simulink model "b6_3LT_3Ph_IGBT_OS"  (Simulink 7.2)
settings: Solver=ode3  SolverMode=SingleTasking  StartTime=0.0  StopTime=0.1  FixedStep=10e-6  MaxStep=1e-5  RelTol=1e-4  AbsTol=1e-4
PreLoadFcn:
  | INIT_B6_3L_3Ph_IGBT_OS
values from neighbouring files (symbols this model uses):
  C = 10e-3*1    (= 0.01)    [INIT_B6_2L_3Ph_IGBT_OS.m]    (also in INIT_B6_3L_3Ph_IGBT_OS.m; INIT_MMC_100L.m = 0.005; INIT_MMC_200L.m = 0.005; INIT_MMC_20L.m)
  FS = 900    [INIT_B6_2L_3Ph_IGBT_OS.m]    (also in INIT_B6_3L_3Ph_IGBT_OS.m; INIT_PWM_2L.m = 1000; INIT_PWM_3L.m = 1000; INIT_PWM_Con.m = 1000)
  I_B = INS    [INIT_B6_2L_3Ph_IGBT_OS.m]    (also in INIT_B6_3L_3Ph_IGBT_OS.m; INIT_PWM_2L.m = INP; INIT_PWM_3L.m = INP; INIT_PWM_Con.m = INP)
  IDC = PDC/VDC    (= 166.666666667)    [INIT_B6_2L_3Ph_IGBT_OS.m]    (also in INIT_B6_3L_3Ph_IGBT_OS.m = 100; INIT_PWM_2L.m = 16.6666666667; INIT_PWM_3L.m = 83.3333333333; INIT_PWM_Con.m = 83.3333333333)
  LS = 1e-3    (= 0.001)    [INIT_B6_2L_3Ph_IGBT_OS.m]    (also in INIT_B6_3L_3Ph_IGBT_OS.m; INIT_MMC_100L.m = 0.025; INIT_MMC_200L.m = 0.025; INIT_MMC_20L.m = 0.0025)
  UC0 = 600    [INIT_B6_2L_3Ph_IGBT_OS.m]    (also in INIT_B6_3L_3Ph_IGBT_OS.m = 500; INIT_MMC_100L.m = 6800; INIT_MMC_200L.m = 3400; INIT_MMC_20L.m = 5000)
  UNS = ULLP/sqrt(3)    [INIT_B6_2L_3Ph_IGBT_OS.m]    (also in INIT_B6_3L_3Ph_IGBT_OS.m; INIT_MMC_100L.m = ULLP/sqrt(3)*340/400; INIT_MMC_200L.m = ULLP/sqrt(3)*340/400; INIT_MMC_20L.m)

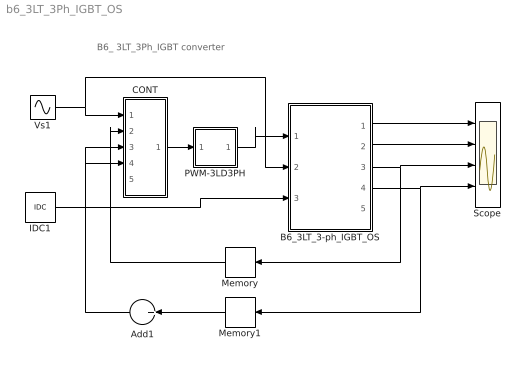
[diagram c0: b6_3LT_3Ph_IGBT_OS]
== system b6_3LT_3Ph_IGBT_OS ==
  note: B6_ 3LT_3Ph_IGBT converter
  Add1 : Sum  Orientation=left  Inputs=+  OutDataType=sfix(16)  OutScaling=2^-10
  B6_3LT_3-ph_IGBT_OS : Subsystem  mask(6-Pulse 3-LT IGBT 3-Phase Converter){LS=LS, C=C, VC0=UC0, RL=1e6}
      mask prompts: LS "Source Inductance"; C "Load Cap"; VC0 "Initial Cap Voltage"; RL "Load Resistance"
      mask help: Input Vector u: u[0]= IGBT1.gate u[1]= IGBT2.gate u[2]= IGBT3.gate u[3]= IGBT4.gate u[4]= IGBT5.gate u[5]= IGBT6.gate u[6]= IGBT7.gate u[7]= IGBT8.gate u[8]= IGBT9.gate u[9]= IGBT10.gate u[10]= IGBT11.gate u[11]= IGBT12.gate u[12]= V1.V u[13]= V2.V u[14]= V3.V u[15]= IDC.i Output Vector y: y[0]= T1.I y[1]= D1.I y[2]= T1.V y[3]= T2.I y[4]= D2.I y[5]= T2.V y[6]= LS1.I y[7]= LS2.I y[8]= LS3.I y[9]= DC1.V y[10]= DC2.V y[11]= Vab.V Parameter Vector p: p[0]= Ls.L p[1]= C1.C p[2]= C1.vC0 p[3]= R1.r You can pause the simulation during running, change the Parameters you want and continue the Simulation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
  CONT : Subsystem
  IDC1 : Constant  Value=IDC
  Memory : Memory  Orientation=left
  Memory1 : Memory  Orientation=left
  PWM-3LD3PH : Subsystem  mask(PWM-3LD3PH){FT=FS, PHT=0, A=0.5, O1=0.5, O2=-0.5, DT=1e-6}
      mask prompts: FT "Frequency of Trian Sig."; PHT "Phase Angle of Trian. Sig."; A "Amplitude of Trian. Sig."; O1 "Offset of 1st Trian"; O2 "Offset of 2nd Trian."; DT "Dead Time"
      mask help: Pulse Width Modulation for 3 Phase 3 Level Neutral point clamped Converter
  Scope : Scope  NumInputPorts=4
  Vs1 : Sin  Amplitude=UNS  Frequency=50*2*pi  Phase="[0  -2*pi/3   -4*pi/3]"  SampleTime=0
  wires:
  Vs1/1 -> CONT/1(UN), B6_3LT_3-ph_IGBT_OS/2(vS)
  IDC1/1 -> CONT/4(Id*), B6_3LT_3-ph_IGBT_OS/3(iDC)
  CONT/1(A) -> PWM-3LD3PH/1(In1)
  PWM-3LD3PH/1(Out1) -> B6_3LT_3-ph_IGBT_OS/1(SWs)
  B6_3LT_3-ph_IGBT_OS/3(iLs123) -> Scope/3, Memory/1
  Memory/1 -> CONT/2(Iwr)
  B6_3LT_3-ph_IGBT_OS/1(iT1,iD1,vT1) -> Scope/1
  B6_3LT_3-ph_IGBT_OS/2(iT2,iD2,vT2) -> Scope/2
  B6_3LT_3-ph_IGBT_OS/4(vDC12) -> Scope/4, Memory1/1
  Memory1/1 -> Add1/1
  Add1/1 -> CONT/3(UDC)

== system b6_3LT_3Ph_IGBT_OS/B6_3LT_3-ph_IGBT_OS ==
  SWs : Inport  OutDataType=sfix(16)  OutScaling=2^0
  vS : Inport  Port=2  OutDataType=sfix(16)  OutScaling=2^0
  iDC : Inport  Port=3  OutDataType=sfix(16)  OutScaling=2^0
  Mux : Mux  Inputs="[12  3  1]"
  b2_IGBT : S-Function  FunctionName=s_b6_3LT_3Ph_IGBT_OS  Parameters="[ LS  C  VC0 RL]"  EnableBusSupport=off
  iT1,iD1,vT1 : Outport  OutDataType=sfix(16)  OutScaling=2^0
  iT2,iD2,vT2 : Outport  Port=2  OutDataType=sfix(16)  OutScaling=2^0
  iLs123 : Outport  Port=3  OutDataType=sfix(16)  OutScaling=2^0
  vDC12 : Outport  Port=4  OutDataType=sfix(16)  OutScaling=2^0
  vab : Outport  Port=5  OutDataType=sfix(16)  OutScaling=2^0
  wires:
  b2_IGBT/5 -> vab/1
  SWs/1 -> Mux/1
  vS/1 -> Mux/2
  b2_IGBT/1 -> iT1,iD1,vT1/1
  b2_IGBT/2 -> iT2,iD2,vT2/1
  b2_IGBT/3 -> iLs123/1
  iDC/1 -> Mux/3
  Mux/1 -> b2_IGBT/1
  b2_IGBT/4 -> vDC12/1

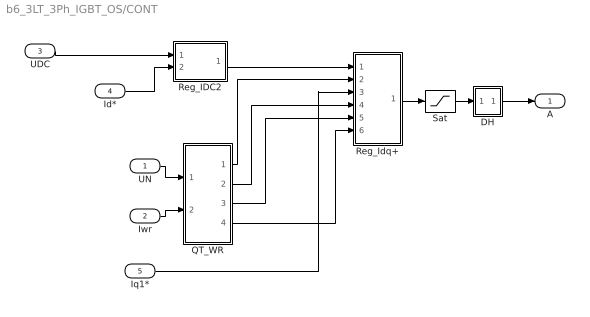
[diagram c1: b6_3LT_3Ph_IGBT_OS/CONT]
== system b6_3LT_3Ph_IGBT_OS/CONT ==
  UN : Inport
  Iwr : Inport  Port=2
  UDC : Inport  Port=3
  Id* : Inport  Port=4
  Iq1* : Inport  Port=5
  DH : Subsystem
  QT_WR : Subsystem
  Reg_IDC2 : Subsystem
  Reg_Idq+ : Subsystem
  Sat : Saturate  UpperLimit=1.5  LowerLimit=-1.5
  A : Outport
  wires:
  Sat/1 -> DH/1(I)
  Reg_Idq+/1(A+) -> Sat/1
  Id*/1 -> Reg_IDC2/2(Id*)
  DH/1(O) -> A/1
  UDC/1 -> Reg_IDC2/1(UDC)
  UN/1 -> QT_WR/1(UN)
  Iwr/1 -> QT_WR/2(I_WR)
  Reg_IDC2/1(Id1*) -> Reg_Idq+/1(Id1*)
  QT_WR/3(th1) -> Reg_Idq+/5(th)
  Iq1*/1 -> Reg_Idq+/3(Iq1*)
  QT_WR/2(Iq1) -> Reg_Idq+/4(Iq1)
  QT_WR/1(Id1) -> Reg_Idq+/2(Id1)
  QT_WR/4(Ud) -> Reg_Idq+/6(Ud)

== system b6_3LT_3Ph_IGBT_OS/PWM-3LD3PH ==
  In1 : Inport  OutDataType=sfix(16)  OutScaling=2^0
  Demux1 : Demux  Outputs=3
  Mux1 : Mux  Inputs=3
  PWM-3LD1PH : Subsystem  mask(PWM-3LD_1PH){FT=FT, PHT=PHT, A=A, O1=O1, O2=O2, DT=DT}
      mask prompts: FT "Frequency of Trian Sig."; PHT "Phase Angle of Trian. Sig."; A "Amplitude of Trian. Sig."; O1 "Offset of 1st Trian"; O2 "Offset of 2nd Trian."; DT "Dead Time"
      mask help: Pulse Width Modulation for 1 Leg of 3 Level Neutral point clamped Converter
  PWM-3LD1PH1 : Subsystem  mask(PWM-3LD_1PH){FT=FT, PHT=PHT, A=A, O1=O1, O2=O2, DT=DT}
      mask prompts: FT "Frequency of Trian Sig."; PHT "Phase Angle of Trian. Sig."; A "Amplitude of Trian. Sig."; O1 "Offset of 1st Trian"; O2 "Offset of 2nd Trian."; DT "Dead Time"
      mask help: Pulse Width Modulation for 1 Leg of 3 Level Neutral point clamped Converter
  PWM-3LD1PH2 : Subsystem  mask(PWM-3LD_1PH){FT=FT, PHT=PHT, A=A, O1=O1, O2=O2, DT=DT}
      mask prompts: FT "Frequency of Trian Sig."; PHT "Phase Angle of Trian. Sig."; A "Amplitude of Trian. Sig."; O1 "Offset of 1st Trian"; O2 "Offset of 2nd Trian."; DT "Dead Time"
      mask help: Pulse Width Modulation for 1 Leg of 3 Level Neutral point clamped Converter
  Out1 : Outport
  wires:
  In1/1 -> Demux1/1
  Demux1/3 -> PWM-3LD1PH2/1(In1)
  Demux1/2 -> PWM-3LD1PH1/1(In1)
  Demux1/1 -> PWM-3LD1PH/1(In1)
  Mux1/1 -> Out1/1
  PWM-3LD1PH2/1(Out1) -> Mux1/3
  PWM-3LD1PH1/1(Out1) -> Mux1/2
  PWM-3LD1PH/1(Out1) -> Mux1/1

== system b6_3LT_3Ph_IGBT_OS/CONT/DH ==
  I : Inport
  Gain : Gain  Gain=0.5
  MinMax : MinMax
  MinMax1 : MinMax  Function=max
  Sum6 : Sum  Inputs=--
  Sum7 : Sum
  O : Outport  InitialOutput=0
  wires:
  I/1 -> MinMax1/1, MinMax/1, Sum7/1
  MinMax/1 -> Sum6/1
  MinMax1/1 -> Sum6/2
  Sum6/1 -> Gain/1
  Gain/1 -> Sum7/2
  Sum7/1 -> O/1

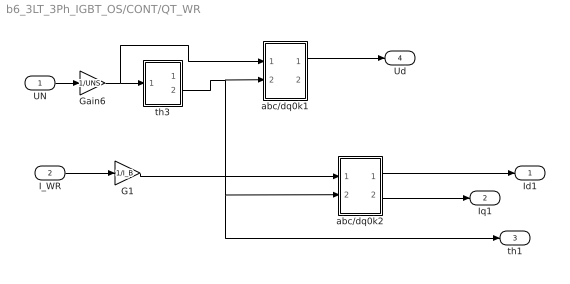
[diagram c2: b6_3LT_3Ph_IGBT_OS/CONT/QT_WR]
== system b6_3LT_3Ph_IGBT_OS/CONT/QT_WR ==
  UN : Inport
  I_WR : Inport  Port=2
  G1 : Gain  Gain=1/I_B
  Gain6 : Gain  Gain=1/UNS
  abc/dq0k1 : Subsystem
  abc/dq0k2 : Subsystem
  th3 : Subsystem
  Id1 : Outport
  Iq1 : Outport  Port=2
  th1 : Outport  Port=3
  Ud : Outport  Port=4
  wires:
  th3/2(th) -> abc/dq0k2/2(th), th1/1, abc/dq0k1/2(th)
  I_WR/1 -> G1/1
  G1/1 -> abc/dq0k2/1(a)
  UN/1 -> Gain6/1
  Gain6/1 -> th3/1(abc), abc/dq0k1/1(a)
  abc/dq0k2/1(dk) -> Id1/1
  abc/dq0k2/2(qk) -> Iq1/1
  abc/dq0k1/1(dk) -> Ud/1

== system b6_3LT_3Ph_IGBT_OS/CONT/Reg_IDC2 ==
  UDC : Inport
  Id* : Inport  Port=2
  Add : Sum
  G1 : Gain  Gain=1/IDC
  G4 : Gain  Gain=1/2/UC0
  PIC : Subsystem  mask(PI-controller){Kp=2, Ki=10, lim=2, Ts=-1}
      mask prompts: Kp "Proportional gain (Kp)"; Ki "Integral gain (Ki)"; lim "Output limit"; Ts "Sampling time (s)"
      mask help: Proportional-Integral Controller
  Sat : Saturate  UpperLimit=2  LowerLimit=-2
  UDC* : Constant  Value=1.0
  Id1* : Outport
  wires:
  Id*/1 -> G1/1
  PIC/1(e*) -> Add/2
  Sat/1 -> Id1*/1
  Add/1 -> Sat/1
  G4/1 -> PIC/2(c)
  UDC*/1 -> PIC/1(c*)
  UDC/1 -> G4/1
  G1/1 -> Add/1

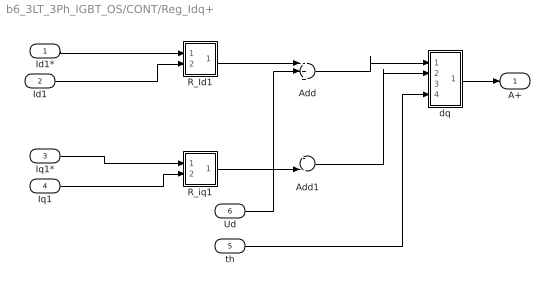
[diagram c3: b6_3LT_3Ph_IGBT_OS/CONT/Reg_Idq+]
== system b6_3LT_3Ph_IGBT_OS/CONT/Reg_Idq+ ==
  Id1* : Inport
  Id1 : Inport  Port=2
  Iq1* : Inport  Port=3
  Iq1 : Inport  Port=4
  th : Inport  Port=5
  Ud : Inport  Port=6
  Add : Sum  Inputs=-++
  Add1 : Sum  Inputs=--
  R_Id1 : Subsystem  mask(PI-controller){Kp=0.1, Ki=200, lim=2, Ts=-1}
      mask prompts: Kp "Proportional gain (Kp)"; Ki "Integral gain (Ki)"; lim "Output limit"; Ts "Sampling time (s)"
      mask help: Proportional-Integral Controller
  R_iq1 : Subsystem  mask(PI-controller){Kp=0.1, Ki=200, lim=2, Ts=-2}
      mask prompts: Kp "Proportional gain (Kp)"; Ki "Integral gain (Ki)"; lim "Output limit"; Ts "Sampling time (s)"
      mask help: Proportional-Integral Controller
  dq : Subsystem
  A+ : Outport
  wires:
  Iq1/1 -> R_iq1/2(c)
  Iq1*/1 -> R_iq1/1(c*)
  Id1/1 -> R_Id1/2(c)
  Id1*/1 -> R_Id1/1(c*)
  dq/1(a) -> A+/1
  th/1 -> dq/4(th)
  R_Id1/1(e*) -> Add/1
  R_iq1/1(e*) -> Add1/2
  Add/1 -> dq/1(dk)
  Add1/1 -> dq/2(qk)
  Ud/1 -> Add/2

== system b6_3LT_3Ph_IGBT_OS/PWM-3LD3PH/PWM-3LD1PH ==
  In1 : Inport  OutDataType=sfix(16)  OutScaling=2^0
  Mux : Mux
  SS : Subsystem
  SS1 : Subsystem
  Out1 : Outport
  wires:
  In1/1 -> SS1/1(I1), SS/1(I1)
  SS1/1(O1) -> Mux/2
  SS/2(O2) -> Mux/3
  Mux/1 -> Out1/1
  SS/1(O1) -> Mux/1
  SS1/2(O2) -> Mux/4

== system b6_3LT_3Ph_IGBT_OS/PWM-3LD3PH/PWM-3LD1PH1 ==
  In1 : Inport  OutDataType=sfix(16)  OutScaling=2^0
  Mux : Mux
  SS : Subsystem
  SS1 : Subsystem
  Out1 : Outport
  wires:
  SS1/2(O2) -> Mux/4
  SS/1(O1) -> Mux/1
  Mux/1 -> Out1/1
  SS/2(O2) -> Mux/3
  SS1/1(O1) -> Mux/2
  In1/1 -> SS/1(I1), SS1/1(I1)

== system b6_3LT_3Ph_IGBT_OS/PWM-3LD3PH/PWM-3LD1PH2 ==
  In1 : Inport  OutDataType=sfix(16)  OutScaling=2^0
  Mux : Mux
  SS : Subsystem
  SS1 : Subsystem
  Out1 : Outport
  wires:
  In1/1 -> SS1/1(I1), SS/1(I1)
  SS1/1(O1) -> Mux/2
  SS/2(O2) -> Mux/3
  Mux/1 -> Out1/1
  SS/1(O1) -> Mux/1
  SS1/2(O2) -> Mux/4

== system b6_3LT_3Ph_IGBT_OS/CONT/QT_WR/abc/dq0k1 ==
  a : Inport
  th : Inport  Port=2
  Demux : Demux  Outputs=3
  Fcn : Fcn  Expr=u(1)*cos(u(3)) + u(2)*sin(u(3))
  Fcn1 : Fcn  Expr=-u(1)*sin(u(3)) + u(2)*cos(u(3))
  K : Gain  Gain="2/3*[1   -.5   -.5;  0   sqrt(3)/2   -sqrt(3)/2;  .5    .5    .5]"  Multiplication=Matrix(K*u)
  Mux1 : Mux  Inputs=3
  dk : Outport
  qk : Outport  Port=2
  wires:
  Demux/2 -> Mux1/2
  Demux/1 -> Mux1/1
  th/1 -> Mux1/3
  Fcn1/1 -> qk/1
  Fcn/1 -> dk/1
  Mux1/1 -> Fcn/1, Fcn1/1
  a/1 -> K/1
  K/1 -> Demux/1

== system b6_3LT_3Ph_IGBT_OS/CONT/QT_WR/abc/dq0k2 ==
  a : Inport
  th : Inport  Port=2
  Demux : Demux  Outputs=3
  Fcn : Fcn  Expr=u(1)*cos(u(3)) + u(2)*sin(u(3))
  Fcn1 : Fcn  Expr=-u(1)*sin(u(3)) + u(2)*cos(u(3))
  K : Gain  Gain="2/3*[1   -.5   -.5;  0   sqrt(3)/2   -sqrt(3)/2;  .5    .5    .5]"  Multiplication=Matrix(K*u)
  Mux1 : Mux  Inputs=3
  dk : Outport
  qk : Outport  Port=2
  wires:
  K/1 -> Demux/1
  a/1 -> K/1
  Mux1/1 -> Fcn1/1, Fcn/1
  Fcn/1 -> dk/1
  Fcn1/1 -> qk/1
  th/1 -> Mux1/3
  Demux/1 -> Mux1/1
  Demux/2 -> Mux1/2

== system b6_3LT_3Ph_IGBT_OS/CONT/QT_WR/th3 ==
  abc : Inport
  C : ComplexToMagnitudeAngle
  Demux : Demux  Outputs=3
  K : Gain  Gain="2/3*[1   -.5   -.5;  0   sqrt(3)/2   -sqrt(3)/2;  .5    .5    .5]"  Multiplication=Matrix(K*u)
  R : RealImagToComplex
  |u| : Outport
  th : Outport  Port=2
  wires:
  C/2 -> th/1
  R/1 -> C/1
  Demux/2 -> R/2
  Demux/1 -> R/1
  abc/1 -> K/1
  K/1 -> Demux/1
  C/1 -> |u|/1

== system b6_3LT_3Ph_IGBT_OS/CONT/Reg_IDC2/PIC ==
  c* : Inport  OutDataType=sfix(16)  OutScaling=2^0
  c : Inport  Port=2  OutDataType=sfix(16)  OutScaling=2^0
  Gain : Gain  Gain=Ki  ParameterDataType=sfix(16)  ParameterScaling=2^0  OutDataType=sfix(16)  OutScaling=2^0
  Gain1 : Gain  Gain=Kp  ParameterDataType=sfix(16)  ParameterScaling=2^0  OutDataType=sfix(16)  OutScaling=2^0
  Integrator : Integrator  UpperSaturationLimit=lim  LowerSaturationLimit=-lim
  Saturation : Saturate  UpperLimit=lim  LowerLimit=-lim
  Sum1 : Sum  Inputs=+-  OutDataType=sfix(16)  OutScaling=2^0
  Sum2 : Sum  OutDataType=sfix(16)  OutScaling=2^0
  e* : Outport  InitialOutput=0
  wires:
  Integrator/1 -> Sum2/2
  c*/1 -> Sum1/1
  c/1 -> Sum1/2
  Saturation/1 -> e*/1
  Sum2/1 -> Saturation/1
  Sum1/1 -> Gain1/1, Gain/1
  Gain1/1 -> Sum2/1
  Gain/1 -> Integrator/1

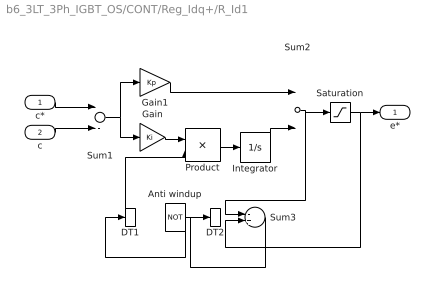
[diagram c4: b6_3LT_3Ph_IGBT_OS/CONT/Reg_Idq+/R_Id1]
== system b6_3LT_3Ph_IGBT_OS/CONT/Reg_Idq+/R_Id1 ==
  c* : Inport
  c : Inport  Port=2
  Anti windup : Logic  Operator=NOT
  DT1 : DataTypeConversion
  DT2 : DataTypeConversion
  Gain : Gain  Gain=Ki
  Gain1 : Gain  Gain=Kp
  Integrator : Integrator  UpperSaturationLimit=lim  LowerSaturationLimit=-lim
  Product : Product
  Saturation : Saturate  UpperLimit=lim  LowerLimit=-lim
  Sum1 : Sum  Inputs=+-
  Sum2 : Sum
  Sum3 : Sum  Inputs=-+
  e* : Outport  InitialOutput=0
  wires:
  Integrator/1 -> Sum2/2
  c*/1 -> Sum1/1
  c/1 -> Sum1/2
  Saturation/1 -> e*/1, Sum3/2
  Sum2/1 -> Saturation/1, Sum3/1
  Sum1/1 -> Gain1/1, Gain/1
  Gain1/1 -> Sum2/1
  Anti windup/1 -> DT1/1
  DT1/1 -> Product/2
  Gain/1 -> Product/1
  Product/1 -> Integrator/1
  DT2/1 -> Anti windup/1
  Sum3/1 -> DT2/1

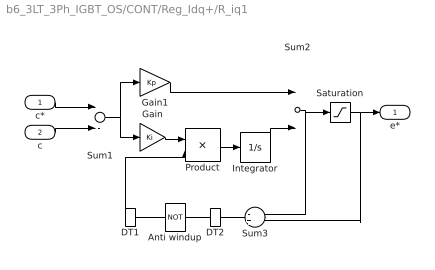
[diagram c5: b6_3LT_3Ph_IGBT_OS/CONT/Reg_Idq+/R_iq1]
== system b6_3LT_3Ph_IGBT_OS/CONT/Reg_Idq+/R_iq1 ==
  c* : Inport
  c : Inport  Port=2
  Anti windup : Logic  Operator=NOT
  DT1 : DataTypeConversion
  DT2 : DataTypeConversion
  Gain : Gain  Gain=Ki
  Gain1 : Gain  Gain=Kp
  Integrator : Integrator  UpperSaturationLimit=lim  LowerSaturationLimit=-lim
  Product : Product
  Saturation : Saturate  UpperLimit=lim  LowerLimit=-lim
  Sum1 : Sum  Inputs=+-
  Sum2 : Sum
  Sum3 : Sum  Inputs=-+
  e* : Outport  InitialOutput=0
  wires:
  Sum3/1 -> DT2/1
  DT2/1 -> Anti windup/1
  Product/1 -> Integrator/1
  Gain/1 -> Product/1
  DT1/1 -> Product/2
  Anti windup/1 -> DT1/1
  Gain1/1 -> Sum2/1
  Sum1/1 -> Gain/1, Gain1/1
  Sum2/1 -> Sum3/1, Saturation/1
  Saturation/1 -> Sum3/2, e*/1
  c/1 -> Sum1/2
  c*/1 -> Sum1/1
  Integrator/1 -> Sum2/2

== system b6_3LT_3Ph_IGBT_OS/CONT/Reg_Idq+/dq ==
  dk : Inport
  qk : Inport  Port=2
  0k : Inport  Port=3
  th : Inport  Port=4
  Fcn : Fcn  Expr=u(1)*cos(u(3)) - u(2)*sin(u(3))
  Fcn1 : Fcn  Expr=u(1)*sin(u(3)) + u(2)*cos(u(3))
  K : Gain  Gain="[1   0  1 ;  -.5   sqrt(3)/2    1 ;  -.5    -sqrt(3)/2    1]"  Multiplication=Matrix(K*u)
  Mux : Mux  Inputs=3
  Mux1 : Mux  Inputs=3
  a : Outport
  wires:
  0k/1 -> Mux1/3
  th/1 -> Mux/3
  Fcn1/1 -> Mux1/2
  Fcn/1 -> Mux1/1
  Mux1/1 -> K/1
  K/1 -> a/1
  Mux/1 -> Fcn1/1, Fcn/1
  qk/1 -> Mux/2
  dk/1 -> Mux/1

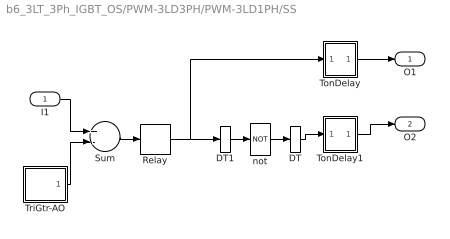
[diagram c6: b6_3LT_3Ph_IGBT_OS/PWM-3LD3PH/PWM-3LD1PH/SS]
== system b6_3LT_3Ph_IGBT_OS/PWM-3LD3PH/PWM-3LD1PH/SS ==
  I1 : Inport  OutDataType=sfix(16)  OutScaling=2^0
  DT : DataTypeConversion
  DT1 : DataTypeConversion
  Relay : Relay  OutDataType=sfix(16)  OutScaling=2^0
  Sum : Sum  Inputs=+-  OutDataType=sfix(16)  OutScaling=2^0
  TonDelay : Subsystem  mask(TonDelay){DT=DT}
      mask prompts: DT "Dead Time"
      mask help: Turn on dead time to protect against short circuit of the converter leg
  TonDelay1 : Subsystem  mask(TonDelay){DT=DT}
      mask prompts: DT "Dead Time"
      mask help: Turn on dead time to protect against short circuit of the converter leg
  TriGtr-AO : Subsystem  mask(TriGtr-AO){A=A, O=O1, T=1/FT, Td=PHT/FT/180}
      mask prompts: A "Amplitude"; O "Offset"; T "Period Time"; Td "Time Delay"
      mask help: Triangular Wave Generator with variable time delay, variable amplitude and offset
  not : Logic  Operator=NOT  Inputs=1
  O1 : Outport  InitialOutput=0
  O2 : Outport  Port=2  InitialOutput=0
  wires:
  TonDelay/1(s1d) -> O1/1
  Relay/1 -> TonDelay/1(s1), DT1/1
  TonDelay1/1(s1d) -> O2/1
  not/1 -> DT/1
  Sum/1 -> Relay/1
  TriGtr-AO/1(Out1) -> Sum/2
  I1/1 -> Sum/1
  DT/1 -> TonDelay1/1(s1)
  DT1/1 -> not/1

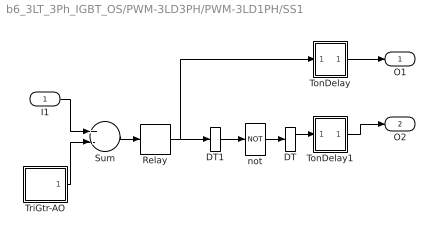
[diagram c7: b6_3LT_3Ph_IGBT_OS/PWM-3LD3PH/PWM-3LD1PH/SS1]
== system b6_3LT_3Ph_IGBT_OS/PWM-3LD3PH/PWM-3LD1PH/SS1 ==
  I1 : Inport  OutDataType=sfix(16)  OutScaling=2^0
  DT : DataTypeConversion
  DT1 : DataTypeConversion
  Relay : Relay  OutDataType=sfix(16)  OutScaling=2^0
  Sum : Sum  Inputs=+-  OutDataType=sfix(16)  OutScaling=2^0
  TonDelay : Subsystem  mask(TonDelay){DT=DT}
      mask prompts: DT "Dead Time"
      mask help: Turn on dead time to protect against short circuit of the converter leg
  TonDelay1 : Subsystem  mask(TonDelay){DT=DT}
      mask prompts: DT "Dead Time"
      mask help: Turn on dead time to protect against short circuit of the converter leg
  TriGtr-AO : Subsystem  mask(TriGtr-AO){A=A, O=O2, T=1/FT, Td=PHT/FT/180}
      mask prompts: A "Amplitude"; O "Offset"; T "Period Time"; Td "Time Delay"
      mask help: Triangular Wave Generator with variable time delay, variable amplitude and offset
  not : Logic  Operator=NOT  Inputs=1
  O1 : Outport  InitialOutput=0
  O2 : Outport  Port=2  InitialOutput=0
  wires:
  TonDelay/1(s1d) -> O1/1
  Relay/1 -> TonDelay/1(s1), DT1/1
  TonDelay1/1(s1d) -> O2/1
  not/1 -> DT/1
  Sum/1 -> Relay/1
  TriGtr-AO/1(Out1) -> Sum/2
  I1/1 -> Sum/1
  DT/1 -> TonDelay1/1(s1)
  DT1/1 -> not/1

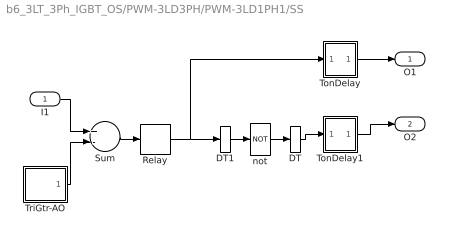
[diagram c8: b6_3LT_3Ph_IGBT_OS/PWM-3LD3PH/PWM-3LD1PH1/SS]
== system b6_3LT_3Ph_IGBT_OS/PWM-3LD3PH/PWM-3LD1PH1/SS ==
  I1 : Inport  OutDataType=sfix(16)  OutScaling=2^0
  DT : DataTypeConversion
  DT1 : DataTypeConversion
  Relay : Relay  OutDataType=sfix(16)  OutScaling=2^0
  Sum : Sum  Inputs=+-  OutDataType=sfix(16)  OutScaling=2^0
  TonDelay : Subsystem  mask(TonDelay){DT=DT}
      mask prompts: DT "Dead Time"
      mask help: Turn on dead time to protect against short circuit of the converter leg
  TonDelay1 : Subsystem  mask(TonDelay){DT=DT}
      mask prompts: DT "Dead Time"
      mask help: Turn on dead time to protect against short circuit of the converter leg
  TriGtr-AO : Subsystem  mask(TriGtr-AO){A=A, O=O1, T=1/FT, Td=PHT/FT/180}
      mask prompts: A "Amplitude"; O "Offset"; T "Period Time"; Td "Time Delay"
      mask help: Triangular Wave Generator with variable time delay, variable amplitude and offset
  not : Logic  Operator=NOT  Inputs=1
  O1 : Outport  InitialOutput=0
  O2 : Outport  Port=2  InitialOutput=0
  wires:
  DT1/1 -> not/1
  DT/1 -> TonDelay1/1(s1)
  I1/1 -> Sum/1
  TriGtr-AO/1(Out1) -> Sum/2
  Sum/1 -> Relay/1
  not/1 -> DT/1
  TonDelay1/1(s1d) -> O2/1
  Relay/1 -> DT1/1, TonDelay/1(s1)
  TonDelay/1(s1d) -> O1/1

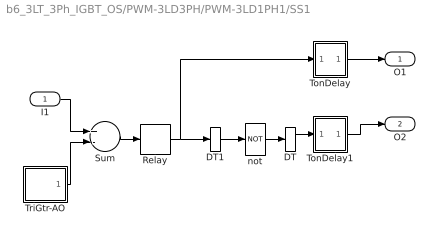
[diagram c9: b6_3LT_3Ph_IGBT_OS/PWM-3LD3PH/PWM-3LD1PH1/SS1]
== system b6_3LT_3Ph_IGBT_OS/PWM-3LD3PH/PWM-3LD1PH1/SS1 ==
  I1 : Inport  OutDataType=sfix(16)  OutScaling=2^0
  DT : DataTypeConversion
  DT1 : DataTypeConversion
  Relay : Relay  OutDataType=sfix(16)  OutScaling=2^0
  Sum : Sum  Inputs=+-  OutDataType=sfix(16)  OutScaling=2^0
  TonDelay : Subsystem  mask(TonDelay){DT=DT}
      mask prompts: DT "Dead Time"
      mask help: Turn on dead time to protect against short circuit of the converter leg
  TonDelay1 : Subsystem  mask(TonDelay){DT=DT}
      mask prompts: DT "Dead Time"
      mask help: Turn on dead time to protect against short circuit of the converter leg
  TriGtr-AO : Subsystem  mask(TriGtr-AO){A=A, O=O2, T=1/FT, Td=PHT/FT/180}
      mask prompts: A "Amplitude"; O "Offset"; T "Period Time"; Td "Time Delay"
      mask help: Triangular Wave Generator with variable time delay, variable amplitude and offset
  not : Logic  Operator=NOT  Inputs=1
  O1 : Outport  InitialOutput=0
  O2 : Outport  Port=2  InitialOutput=0
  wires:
  DT1/1 -> not/1
  DT/1 -> TonDelay1/1(s1)
  I1/1 -> Sum/1
  TriGtr-AO/1(Out1) -> Sum/2
  Sum/1 -> Relay/1
  not/1 -> DT/1
  TonDelay1/1(s1d) -> O2/1
  Relay/1 -> DT1/1, TonDelay/1(s1)
  TonDelay/1(s1d) -> O1/1

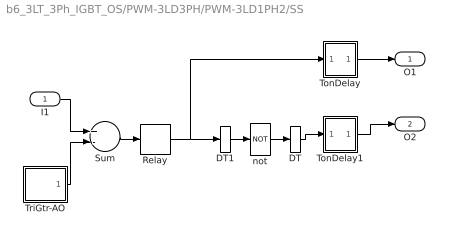
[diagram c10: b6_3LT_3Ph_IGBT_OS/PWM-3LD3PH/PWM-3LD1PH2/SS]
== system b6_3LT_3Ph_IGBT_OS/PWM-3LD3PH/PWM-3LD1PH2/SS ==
  I1 : Inport  OutDataType=sfix(16)  OutScaling=2^0
  DT : DataTypeConversion
  DT1 : DataTypeConversion
  Relay : Relay  OutDataType=sfix(16)  OutScaling=2^0
  Sum : Sum  Inputs=+-  OutDataType=sfix(16)  OutScaling=2^0
  TonDelay : Subsystem  mask(TonDelay){DT=DT}
      mask prompts: DT "Dead Time"
      mask help: Turn on dead time to protect against short circuit of the converter leg
  TonDelay1 : Subsystem  mask(TonDelay){DT=DT}
      mask prompts: DT "Dead Time"
      mask help: Turn on dead time to protect against short circuit of the converter leg
  TriGtr-AO : Subsystem  mask(TriGtr-AO){A=A, O=O1, T=1/FT, Td=PHT/FT/180}
      mask prompts: A "Amplitude"; O "Offset"; T "Period Time"; Td "Time Delay"
      mask help: Triangular Wave Generator with variable time delay, variable amplitude and offset
  not : Logic  Operator=NOT  Inputs=1
  O1 : Outport  InitialOutput=0
  O2 : Outport  Port=2  InitialOutput=0
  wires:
  TonDelay/1(s1d) -> O1/1
  Relay/1 -> TonDelay/1(s1), DT1/1
  TonDelay1/1(s1d) -> O2/1
  not/1 -> DT/1
  Sum/1 -> Relay/1
  TriGtr-AO/1(Out1) -> Sum/2
  I1/1 -> Sum/1
  DT/1 -> TonDelay1/1(s1)
  DT1/1 -> not/1

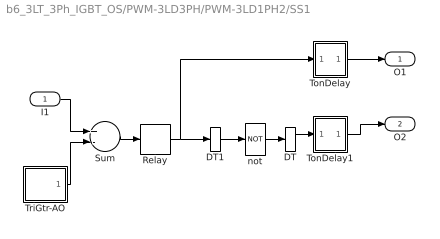
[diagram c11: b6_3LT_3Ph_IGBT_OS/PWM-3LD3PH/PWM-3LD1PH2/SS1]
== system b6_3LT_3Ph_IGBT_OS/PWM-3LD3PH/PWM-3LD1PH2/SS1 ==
  I1 : Inport  OutDataType=sfix(16)  OutScaling=2^0
  DT : DataTypeConversion
  DT1 : DataTypeConversion
  Relay : Relay  OutDataType=sfix(16)  OutScaling=2^0
  Sum : Sum  Inputs=+-  OutDataType=sfix(16)  OutScaling=2^0
  TonDelay : Subsystem  mask(TonDelay){DT=DT}
      mask prompts: DT "Dead Time"
      mask help: Turn on dead time to protect against short circuit of the converter leg
  TonDelay1 : Subsystem  mask(TonDelay){DT=DT}
      mask prompts: DT "Dead Time"
      mask help: Turn on dead time to protect against short circuit of the converter leg
  TriGtr-AO : Subsystem  mask(TriGtr-AO){A=A, O=O2, T=1/FT, Td=PHT/FT/180}
      mask prompts: A "Amplitude"; O "Offset"; T "Period Time"; Td "Time Delay"
      mask help: Triangular Wave Generator with variable time delay, variable amplitude and offset
  not : Logic  Operator=NOT  Inputs=1
  O1 : Outport  InitialOutput=0
  O2 : Outport  Port=2  InitialOutput=0
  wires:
  TonDelay/1(s1d) -> O1/1
  Relay/1 -> TonDelay/1(s1), DT1/1
  TonDelay1/1(s1d) -> O2/1
  not/1 -> DT/1
  Sum/1 -> Relay/1
  TriGtr-AO/1(Out1) -> Sum/2
  I1/1 -> Sum/1
  DT/1 -> TonDelay1/1(s1)
  DT1/1 -> not/1

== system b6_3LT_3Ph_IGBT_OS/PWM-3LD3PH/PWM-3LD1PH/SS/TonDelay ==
  s1 : Inport  Orientation=down  OutDataType=sfix(16)  OutScaling=2^0
  Int : Integrator  ExternalReset=falling
  Rel1 : Relay  OnSwitchValue=DT  OutDataType=sfix(16)  OutScaling=2^0
  s1d : Outport  InitialOutput=0
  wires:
  Rel1/1 -> s1d/1
  s1/1 -> Int/1, Int/2
  Int/1 -> Rel1/1

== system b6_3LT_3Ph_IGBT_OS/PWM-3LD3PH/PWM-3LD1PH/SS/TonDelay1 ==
  s1 : Inport  Orientation=down  OutDataType=sfix(16)  OutScaling=2^0
  Int : Integrator  ExternalReset=falling
  Rel1 : Relay  OnSwitchValue=DT  OutDataType=sfix(16)  OutScaling=2^0
  s1d : Outport  InitialOutput=0
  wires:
  Rel1/1 -> s1d/1
  s1/1 -> Int/1, Int/2
  Int/1 -> Rel1/1

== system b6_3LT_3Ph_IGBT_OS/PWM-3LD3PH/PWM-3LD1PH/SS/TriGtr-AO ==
  Ampl. : Gain  Gain=A  ParameterDataType=sfix(16)  ParameterScaling=2^0  OutDataType=sfix(16)  OutScaling=2^0
  Offset : Constant  Value=O  OutDataType=sfix(16)  OutScaling=2^0
  Sum : Sum  OutDataType=sfix(16)  OutScaling=2^0
  TriGtr1 : Subsystem  mask(TriGtr){T=T, Td=Td}
      mask prompts: T "Period Time"; Td "Time Delay"
      mask help: Triangular Wave Generator with variable time delay
  Out1 : Outport
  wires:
  Sum/1 -> Out1/1
  Ampl./1 -> Sum/1
  TriGtr1/1(O) -> Ampl./1
  Offset/1 -> Sum/2

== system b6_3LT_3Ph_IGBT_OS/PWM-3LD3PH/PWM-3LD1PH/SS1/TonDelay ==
  s1 : Inport  Orientation=down  OutDataType=sfix(16)  OutScaling=2^0
  Int : Integrator  ExternalReset=falling
  Rel1 : Relay  OnSwitchValue=DT  OutDataType=sfix(16)  OutScaling=2^0
  s1d : Outport  InitialOutput=0
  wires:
  Rel1/1 -> s1d/1
  s1/1 -> Int/1, Int/2
  Int/1 -> Rel1/1

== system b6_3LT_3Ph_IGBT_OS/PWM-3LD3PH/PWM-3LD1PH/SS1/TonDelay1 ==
  s1 : Inport  Orientation=down  OutDataType=sfix(16)  OutScaling=2^0
  Int : Integrator  ExternalReset=falling
  Rel1 : Relay  OnSwitchValue=DT  OutDataType=sfix(16)  OutScaling=2^0
  s1d : Outport  InitialOutput=0
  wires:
  Rel1/1 -> s1d/1
  s1/1 -> Int/1, Int/2
  Int/1 -> Rel1/1

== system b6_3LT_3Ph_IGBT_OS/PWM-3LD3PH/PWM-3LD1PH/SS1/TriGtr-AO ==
  Ampl. : Gain  Gain=A  ParameterDataType=sfix(16)  ParameterScaling=2^0  OutDataType=sfix(16)  OutScaling=2^0
  Offset : Constant  Value=O  OutDataType=sfix(16)  OutScaling=2^0
  Sum : Sum  OutDataType=sfix(16)  OutScaling=2^0
  TriGtr1 : Subsystem  mask(TriGtr){T=T, Td=Td}
      mask prompts: T "Period Time"; Td "Time Delay"
      mask help: Triangular Wave Generator with variable time delay
  Out1 : Outport
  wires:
  Offset/1 -> Sum/2
  TriGtr1/1(O) -> Ampl./1
  Ampl./1 -> Sum/1
  Sum/1 -> Out1/1

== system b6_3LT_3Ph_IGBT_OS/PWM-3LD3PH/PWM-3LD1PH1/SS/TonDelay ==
  s1 : Inport  Orientation=down  OutDataType=sfix(16)  OutScaling=2^0
  Int : Integrator  ExternalReset=falling
  Rel1 : Relay  OnSwitchValue=DT  OutDataType=sfix(16)  OutScaling=2^0
  s1d : Outport  InitialOutput=0
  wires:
  Int/1 -> Rel1/1
  s1/1 -> Int/2, Int/1
  Rel1/1 -> s1d/1

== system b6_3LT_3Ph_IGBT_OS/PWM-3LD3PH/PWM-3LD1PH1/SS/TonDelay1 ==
  s1 : Inport  Orientation=down  OutDataType=sfix(16)  OutScaling=2^0
  Int : Integrator  ExternalReset=falling
  Rel1 : Relay  OnSwitchValue=DT  OutDataType=sfix(16)  OutScaling=2^0
  s1d : Outport  InitialOutput=0
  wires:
  Int/1 -> Rel1/1
  s1/1 -> Int/2, Int/1
  Rel1/1 -> s1d/1

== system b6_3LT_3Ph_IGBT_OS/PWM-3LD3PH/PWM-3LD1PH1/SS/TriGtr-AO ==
  Ampl. : Gain  Gain=A  ParameterDataType=sfix(16)  ParameterScaling=2^0  OutDataType=sfix(16)  OutScaling=2^0
  Offset : Constant  Value=O  OutDataType=sfix(16)  OutScaling=2^0
  Sum : Sum  OutDataType=sfix(16)  OutScaling=2^0
  TriGtr1 : Subsystem  mask(TriGtr){T=T, Td=Td}
      mask prompts: T "Period Time"; Td "Time Delay"
      mask help: Triangular Wave Generator with variable time delay
  Out1 : Outport
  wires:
  Offset/1 -> Sum/2
  TriGtr1/1(O) -> Ampl./1
  Ampl./1 -> Sum/1
  Sum/1 -> Out1/1

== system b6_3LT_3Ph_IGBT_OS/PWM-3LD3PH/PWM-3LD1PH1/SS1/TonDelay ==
  s1 : Inport  Orientation=down  OutDataType=sfix(16)  OutScaling=2^0
  Int : Integrator  ExternalReset=falling
  Rel1 : Relay  OnSwitchValue=DT  OutDataType=sfix(16)  OutScaling=2^0
  s1d : Outport  InitialOutput=0
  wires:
  Int/1 -> Rel1/1
  s1/1 -> Int/2, Int/1
  Rel1/1 -> s1d/1

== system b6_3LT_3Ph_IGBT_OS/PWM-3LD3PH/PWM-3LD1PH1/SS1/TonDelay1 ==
  s1 : Inport  Orientation=down  OutDataType=sfix(16)  OutScaling=2^0
  Int : Integrator  ExternalReset=falling
  Rel1 : Relay  OnSwitchValue=DT  OutDataType=sfix(16)  OutScaling=2^0
  s1d : Outport  InitialOutput=0
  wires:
  Int/1 -> Rel1/1
  s1/1 -> Int/2, Int/1
  Rel1/1 -> s1d/1

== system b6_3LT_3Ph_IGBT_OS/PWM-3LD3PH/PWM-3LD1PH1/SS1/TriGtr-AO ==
  Ampl. : Gain  Gain=A  ParameterDataType=sfix(16)  ParameterScaling=2^0  OutDataType=sfix(16)  OutScaling=2^0
  Offset : Constant  Value=O  OutDataType=sfix(16)  OutScaling=2^0
  Sum : Sum  OutDataType=sfix(16)  OutScaling=2^0
  TriGtr1 : Subsystem  mask(TriGtr){T=T, Td=Td}
      mask prompts: T "Period Time"; Td "Time Delay"
      mask help: Triangular Wave Generator with variable time delay
  Out1 : Outport
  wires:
  Sum/1 -> Out1/1
  Ampl./1 -> Sum/1
  TriGtr1/1(O) -> Ampl./1
  Offset/1 -> Sum/2

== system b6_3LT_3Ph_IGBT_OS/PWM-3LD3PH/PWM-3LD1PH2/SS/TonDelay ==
  s1 : Inport  Orientation=down  OutDataType=sfix(16)  OutScaling=2^0
  Int : Integrator  ExternalReset=falling
  Rel1 : Relay  OnSwitchValue=DT  OutDataType=sfix(16)  OutScaling=2^0
  s1d : Outport  InitialOutput=0
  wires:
  Rel1/1 -> s1d/1
  s1/1 -> Int/1, Int/2
  Int/1 -> Rel1/1

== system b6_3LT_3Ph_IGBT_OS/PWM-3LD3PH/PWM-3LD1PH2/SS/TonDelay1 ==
  s1 : Inport  Orientation=down  OutDataType=sfix(16)  OutScaling=2^0
  Int : Integrator  ExternalReset=falling
  Rel1 : Relay  OnSwitchValue=DT  OutDataType=sfix(16)  OutScaling=2^0
  s1d : Outport  InitialOutput=0
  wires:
  Rel1/1 -> s1d/1
  s1/1 -> Int/1, Int/2
  Int/1 -> Rel1/1

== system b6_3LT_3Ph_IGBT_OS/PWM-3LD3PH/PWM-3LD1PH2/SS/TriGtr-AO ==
  Ampl. : Gain  Gain=A  ParameterDataType=sfix(16)  ParameterScaling=2^0  OutDataType=sfix(16)  OutScaling=2^0
  Offset : Constant  Value=O  OutDataType=sfix(16)  OutScaling=2^0
  Sum : Sum  OutDataType=sfix(16)  OutScaling=2^0
  TriGtr1 : Subsystem  mask(TriGtr){T=T, Td=Td}
      mask prompts: T "Period Time"; Td "Time Delay"
      mask help: Triangular Wave Generator with variable time delay
  Out1 : Outport
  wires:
  Sum/1 -> Out1/1
  Ampl./1 -> Sum/1
  TriGtr1/1(O) -> Ampl./1
  Offset/1 -> Sum/2

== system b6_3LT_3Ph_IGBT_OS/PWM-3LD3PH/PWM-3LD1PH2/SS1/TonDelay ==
  s1 : Inport  Orientation=down  OutDataType=sfix(16)  OutScaling=2^0
  Int : Integrator  ExternalReset=falling
  Rel1 : Relay  OnSwitchValue=DT  OutDataType=sfix(16)  OutScaling=2^0
  s1d : Outport  InitialOutput=0
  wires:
  Rel1/1 -> s1d/1
  s1/1 -> Int/1, Int/2
  Int/1 -> Rel1/1

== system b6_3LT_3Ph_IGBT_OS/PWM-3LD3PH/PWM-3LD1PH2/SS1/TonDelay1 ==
  s1 : Inport  Orientation=down  OutDataType=sfix(16)  OutScaling=2^0
  Int : Integrator  ExternalReset=falling
  Rel1 : Relay  OnSwitchValue=DT  OutDataType=sfix(16)  OutScaling=2^0
  s1d : Outport  InitialOutput=0
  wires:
  Rel1/1 -> s1d/1
  s1/1 -> Int/1, Int/2
  Int/1 -> Rel1/1

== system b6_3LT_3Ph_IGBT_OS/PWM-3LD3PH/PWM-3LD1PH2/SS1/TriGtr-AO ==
  Ampl. : Gain  Gain=A  ParameterDataType=sfix(16)  ParameterScaling=2^0  OutDataType=sfix(16)  OutScaling=2^0
  Offset : Constant  Value=O  OutDataType=sfix(16)  OutScaling=2^0
  Sum : Sum  OutDataType=sfix(16)  OutScaling=2^0
  TriGtr1 : Subsystem  mask(TriGtr){T=T, Td=Td}
      mask prompts: T "Period Time"; Td "Time Delay"
      mask help: Triangular Wave Generator with variable time delay
  Out1 : Outport
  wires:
  Offset/1 -> Sum/2
  TriGtr1/1(O) -> Ampl./1
  Ampl./1 -> Sum/1
  Sum/1 -> Out1/1

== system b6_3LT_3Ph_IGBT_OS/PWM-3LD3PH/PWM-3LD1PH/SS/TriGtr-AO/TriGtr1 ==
  Clock : Clock
  S2 : Subsystem
  Sum : Sum  OutDataType=sfix(16)  OutScaling=2^0
  T : Constant  Value=T  OutDataType=sfix(16)  OutScaling=2^0
  Td : Constant  Value=Td  OutDataType=sfix(16)  OutScaling=2^0
  mod : Math  Operator=mod
  O : Outport  InitialOutput=0
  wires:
  Td/1 -> Sum/2
  Sum/1 -> mod/1
  T/1 -> mod/2
  Clock/1 -> Sum/1
  S2/1(O1) -> O/1
  mod/1 -> S2/1(I1)

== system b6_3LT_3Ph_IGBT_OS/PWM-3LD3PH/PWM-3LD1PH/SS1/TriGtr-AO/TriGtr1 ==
  Clock : Clock
  S1 : Subsystem
  Sum : Sum
  T : Constant  Value=T
  Td : Constant  Value=Td
  mod : Math  Operator=mod
  O : Outport  InitialOutput=0
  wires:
  Td/1 -> Sum/2
  Sum/1 -> mod/1
  T/1 -> mod/2
  Clock/1 -> Sum/1
  S1/1(O1) -> O/1
  mod/1 -> S1/1(I1)

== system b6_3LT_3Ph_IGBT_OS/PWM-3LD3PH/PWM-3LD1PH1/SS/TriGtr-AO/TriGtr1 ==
  Clock : Clock
  S2 : Subsystem
  Sum : Sum  OutDataType=sfix(16)  OutScaling=2^0
  T : Constant  Value=T  OutDataType=sfix(16)  OutScaling=2^0
  Td : Constant  Value=Td  OutDataType=sfix(16)  OutScaling=2^0
  mod : Math  Operator=mod
  O : Outport  InitialOutput=0
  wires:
  mod/1 -> S2/1(I1)
  S2/1(O1) -> O/1
  Clock/1 -> Sum/1
  T/1 -> mod/2
  Sum/1 -> mod/1
  Td/1 -> Sum/2

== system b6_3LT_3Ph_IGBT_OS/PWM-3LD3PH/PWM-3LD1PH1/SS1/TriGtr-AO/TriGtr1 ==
  Clock : Clock
  S1 : Subsystem
  Sum : Sum
  T : Constant  Value=T
  Td : Constant  Value=Td
  mod : Math  Operator=mod
  O : Outport  InitialOutput=0
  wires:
  mod/1 -> S1/1(I1)
  S1/1(O1) -> O/1
  Clock/1 -> Sum/1
  T/1 -> mod/2
  Sum/1 -> mod/1
  Td/1 -> Sum/2

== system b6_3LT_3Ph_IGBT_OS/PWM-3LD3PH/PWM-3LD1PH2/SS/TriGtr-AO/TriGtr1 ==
  Clock : Clock
  S2 : Subsystem
  Sum : Sum  OutDataType=sfix(16)  OutScaling=2^0
  T : Constant  Value=T  OutDataType=sfix(16)  OutScaling=2^0
  Td : Constant  Value=Td  OutDataType=sfix(16)  OutScaling=2^0
  mod : Math  Operator=mod
  O : Outport  InitialOutput=0
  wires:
  Td/1 -> Sum/2
  Sum/1 -> mod/1
  T/1 -> mod/2
  Clock/1 -> Sum/1
  S2/1(O1) -> O/1
  mod/1 -> S2/1(I1)

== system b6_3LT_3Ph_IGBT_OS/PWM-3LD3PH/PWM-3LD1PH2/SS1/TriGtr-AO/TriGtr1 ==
  Clock : Clock
  S1 : Subsystem
  Sum : Sum
  T : Constant  Value=T
  Td : Constant  Value=Td
  mod : Math  Operator=mod
  O : Outport  InitialOutput=0
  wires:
  Td/1 -> Sum/2
  Sum/1 -> mod/1
  T/1 -> mod/2
  Clock/1 -> Sum/1
  S1/1(O1) -> O/1
  mod/1 -> S1/1(I1)

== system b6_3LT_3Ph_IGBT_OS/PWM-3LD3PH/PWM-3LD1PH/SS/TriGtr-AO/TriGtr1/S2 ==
  I1 : Inport
  Fcn : Fcn  Expr="(u* (u <=T/4) * 4/T)   +  (  (u > T/4) && ( u <=3*T/4) )* ( 1 - (u-T/4) *4/T )   +  ( (u > 3*T/4)&& (u<=T)) * ( ((u -3*T/4)* 4/T )-1 )"
  O1 : Outport
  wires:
  Fcn/1 -> O1/1
  I1/1 -> Fcn/1

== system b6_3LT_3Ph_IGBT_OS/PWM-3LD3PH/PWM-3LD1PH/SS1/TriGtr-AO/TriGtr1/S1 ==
  I1 : Inport
  Fcn : Fcn  Expr="(u* (u <=T/4) * 4/T)   +  (  (u > T/4) && ( u <=3*T/4) )* ( 1 - (u-T/4) *4/T )   +  ( (u > 3*T/4)&& (u<=T)) * ( ((u -3*T/4)* 4/T )-1 )"
  O1 : Outport
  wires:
  I1/1 -> Fcn/1
  Fcn/1 -> O1/1

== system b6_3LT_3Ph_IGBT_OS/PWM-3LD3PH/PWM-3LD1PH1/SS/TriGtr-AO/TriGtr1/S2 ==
  I1 : Inport
  Fcn : Fcn  Expr="(u* (u <=T/4) * 4/T)   +  (  (u > T/4) && ( u <=3*T/4) )* ( 1 - (u-T/4) *4/T )   +  ( (u > 3*T/4)&& (u<=T)) * ( ((u -3*T/4)* 4/T )-1 )"
  O1 : Outport
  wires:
  I1/1 -> Fcn/1
  Fcn/1 -> O1/1

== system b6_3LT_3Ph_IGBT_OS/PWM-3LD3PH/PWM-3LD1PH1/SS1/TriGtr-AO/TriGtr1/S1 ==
  I1 : Inport
  Fcn : Fcn  Expr="(u* (u <=T/4) * 4/T)   +  (  (u > T/4) && ( u <=3*T/4) )* ( 1 - (u-T/4) *4/T )   +  ( (u > 3*T/4)&& (u<=T)) * ( ((u -3*T/4)* 4/T )-1 )"
  O1 : Outport
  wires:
  Fcn/1 -> O1/1
  I1/1 -> Fcn/1

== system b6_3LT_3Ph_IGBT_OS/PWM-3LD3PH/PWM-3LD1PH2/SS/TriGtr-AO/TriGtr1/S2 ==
  I1 : Inport
  Fcn : Fcn  Expr="(u* (u <=T/4) * 4/T)   +  (  (u > T/4) && ( u <=3*T/4) )* ( 1 - (u-T/4) *4/T )   +  ( (u > 3*T/4)&& (u<=T)) * ( ((u -3*T/4)* 4/T )-1 )"
  O1 : Outport
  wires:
  Fcn/1 -> O1/1
  I1/1 -> Fcn/1

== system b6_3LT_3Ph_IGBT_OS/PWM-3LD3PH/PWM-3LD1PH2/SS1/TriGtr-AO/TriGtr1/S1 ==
  I1 : Inport
  Fcn : Fcn  Expr="(u* (u <=T/4) * 4/T)   +  (  (u > T/4) && ( u <=3*T/4) )* ( 1 - (u-T/4) *4/T )   +  ( (u > 3*T/4)&& (u<=T)) * ( ((u -3*T/4)* 4/T )-1 )"
  O1 : Outport
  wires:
  I1/1 -> Fcn/1
  Fcn/1 -> O1/1
